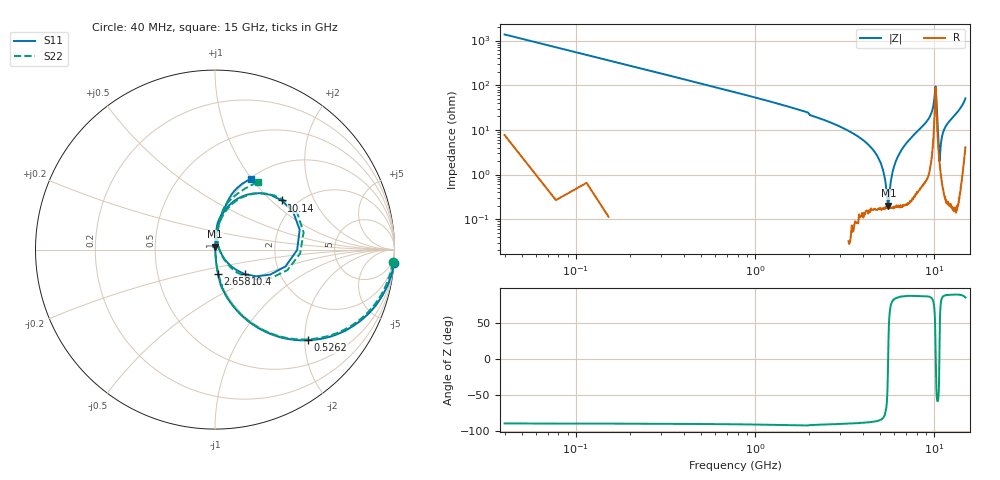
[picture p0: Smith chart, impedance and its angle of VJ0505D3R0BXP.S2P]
! VJ0505D3R0BXP
! MLCC placed on 25 mil thick microstrip substrate in series configuraton.
! DATE 06/29/2018  07:43
! CORRECTED  DATA
# GHz  S  MA  R  50.00
!  FREQ  S11M  S11A  S21M  S21A  S12M  S12A  S22M  S22A
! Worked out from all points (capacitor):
!   401 points, 40 MHz to 15 GHz, reference 50 ohm
!   read as one part in series: C = 2.91 pF near 114.8 MHz
!   lowest |Z| = 200 mohm at 5.575 GHz (marker M1)
!   series resonance near 5.554 GHz, so ESL is about 280 pH
!   S11 on the Smith chart (normalised r, x): 40 MHz: -0, -28; 526.2 MHz: 0.98, -2.08; 2.658 GHz: 1.00, -0.27; 10.14 GHz: 1.68, +1.17; 10.4 GHz: 1.34, -0.39; 15 GHz: 1.01, +0.99
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0.04  1.001 -4.2  0.07304 85.5  0.07384 85.9  0.9935 -4.1
0.227  0.9283 -22.5  0.3838 67.7  0.3839 67.6  0.9202 -22.4
0.5262  0.7243 -44.2  0.6995 46.4  0.6998 46.4  0.7184 -44.1
1.1994  0.4032 -67.5  0.9255 24.1  0.9263 24.1  0.4016 -67.3
2.5458  0.1461 -82.5  0.9912 9.3  0.9917 9.3  0.1462 -81.6
2.658  0.1357 -82.8  0.992 8.8  0.9925 8.8  0.1363 -82.1
4.4906  0.02564 -83.8  0.9973 3.0  0.9981 3.0  0.02546 -84.7
4.8646  0.01072 -78.7  0.9975 2.2  0.9981 2.2  0.01057 -83.6
5.0516  0.003637 -62.3  0.9977 1.9  0.9983 1.9  0.00338 -67.6
5.1638  0.002304 40.9  0.9977 1.6  0.9982 1.6  0.001575 44.3
5.3508  0.008413 79.7  0.9975 1.3  0.9982 1.3  0.008115 81.8
5.5752  0.01688 86.5  0.9974 0.9  0.9978 0.9  0.0169 85.9
6.2858  0.04161 87.5  0.9966 -0.5  0.9972 -0.4  0.04142 87.3
7.52  0.08523 86.3  0.9929 -3.0  0.9936 -2.9  0.0863 84.9
10.0258  0.3756 56.2  0.8287 -19.7  0.83 -19.7  0.3887 53.8
10.138  0.4623 36.4  0.6597 -21.2  0.6607 -21.1  0.4786 33.9
10.3998  0.2166 -39.4  0.8498 11.9  0.8502 12.0  0.2257 -41.7
10.6242  0.03789 -29.7  0.9674 3.1  0.9676 3.1  0.0405 -33.9
10.7364  0.02587 44.4  0.9799 0.9  0.9804 0.9  0.02565 39.3
11.2226  0.09704 85.5  0.9899 -3.9  0.9906 -3.9  0.09904 81.5
12.5316  0.1827 81.0  0.9798 -9.1  0.9808 -9.1  0.1888 79.7
15  0.4423 62.9  0.8611 -25.3  0.8615 -25.3  0.4448 57.5
